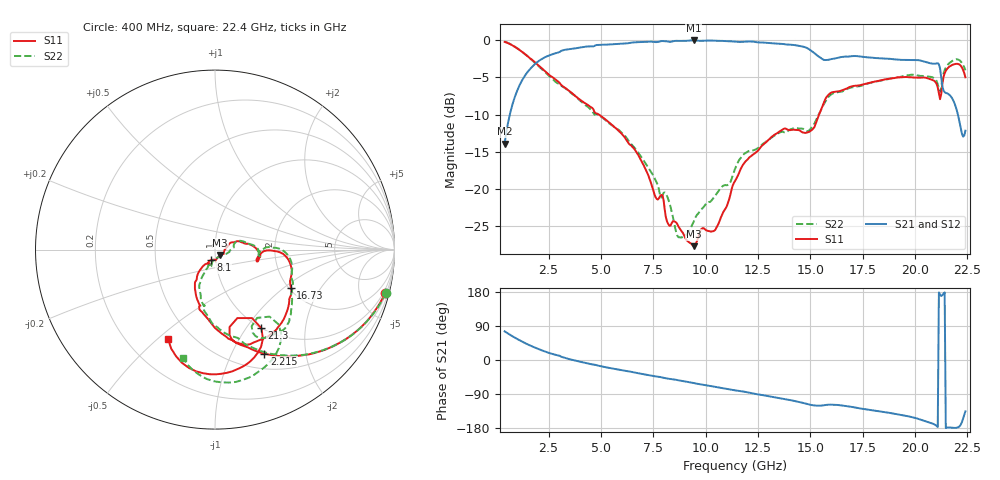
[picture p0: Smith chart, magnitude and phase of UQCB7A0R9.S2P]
!  Part Number  UQCB7A0R9	Mounting Orientation: Vertical
!  Description: RF capacitors
!  Application: Coupling, Bypass, Tuning, DC Block
!  Filters, Matching
# GHZ S DB R 50
! Freq  |S11|  S11 Ph  |S21|  S21 Ph  |S12|  S12 Ph  |S22|  S22 Ph
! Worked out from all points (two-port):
!   401 points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, 400 MHz to 22.4 GHz, reference 50 ohm
!   highest |S21| = -0.01 dB at 9.42 GHz (marker M1); lowest = -13.9 dB at 400 MHz (marker M2)
!   |S21| within 3 dB of the highest: 1.923 GHz to 20.62 GHz (18.69 GHz wide, 166 % of centre)
!   lowest |S11| = -27.8 dB at 9.42 GHz (marker M3), VSWR 1.09, Z = 52.8 - j3.14 ohm
!   |S11| at or under -10 dB: 4.899 GHz to 15.41 GHz (10.51 GHz wide, 104 % of centre)
!   |S22| runs from -26.6 to -0.2 dB; largest |S21 - S12| = 0.0034
!   S11 on the Smith chart (normalised r, x): 400 MHz: 0.72, -7.82; 2.215 GHz: 0.68, -1.34; 8.1 GHz: 0.94, -0.11; 16.73 GHz: 2.05, -1.12; 21.3 GHz: 1.00, -1.18; 22.4 GHz: 0.37, -0.54
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0.4  -0.20 -14.5  -13.94 75.5  -13.94 75.5  -0.17 -14.2
1.115  -1.30 -37.7  -6.04 52.0  -6.04 52.0  -1.28 -37.4
2.215  -3.86 -64.7  -2.44 24.6  -2.44 24.6  -3.97 -64.4
4.085  -8.17 -95.5  -0.92 -5.6  -0.92 -5.6  -8.33 -95.0
6.56  -14.54 -122.7  -0.27 -32.5  -0.27 -32.6  -14.33 -114.5
7.77  -21.28 -108.5  -0.17 -44.3  -0.18 -44.3  -20.12 -112.7
8.1  -23.86 -113.0  -0.12 -48.2  -0.12 -48.2  -20.68 -101.6
8.705  -25.12 -83.5  -0.07 -53.6  -0.07 -53.6  -26.55 -76.6
9.42  -27.75 -46.5  -0.01 -60.6  -0.01 -60.6  -24.50 -25.7
10.52  -25.21 -0.1  -0.05 -71.5  -0.05 -71.5  -20.67 2.4
11.4  -18.97 21.1  -0.17 -80.1  -0.17 -80.1  -17.34 20.2
13.27  -12.75 1.2  -0.41 -98.0  -0.41 -98.0  -12.85 4.3
15.085  -12.04 -6.8  -1.48 -119.2  -1.48 -119.1  -11.64 -0.4
15.855  -7.36 -11.0  -2.62 -118.0  -2.64 -118.1  -7.65 -5.8
16.735  -6.50 -26.7  -2.19 -122.0  -2.20 -121.9  -6.58 -22.5
18.77  -5.16 -48.1  -2.48 -139.5  -2.48 -139.5  -5.17 -39.8
20.035  -5.02 -65.0  -2.65 -153.3  -2.65 -153.3  -4.66 -51.0
21.025  -5.87 -79.4  -3.10 -173.7  -3.10 -173.7  -5.49 -64.9
21.3  -5.86 -59.5  -6.17 171.0  -6.17 171.0  -5.24 -49.6
21.52  -3.87 -70.2  -7.13 -178.6  -7.15 -178.5  -3.43 -59.7
21.905  -3.19 -86.9  -8.68 -179.2  -8.68 -179.1  -2.59 -78.0
22.4  -4.98 -117.6  -12.18 -135.6  -12.26 -135.6  -4.04 -106.5
